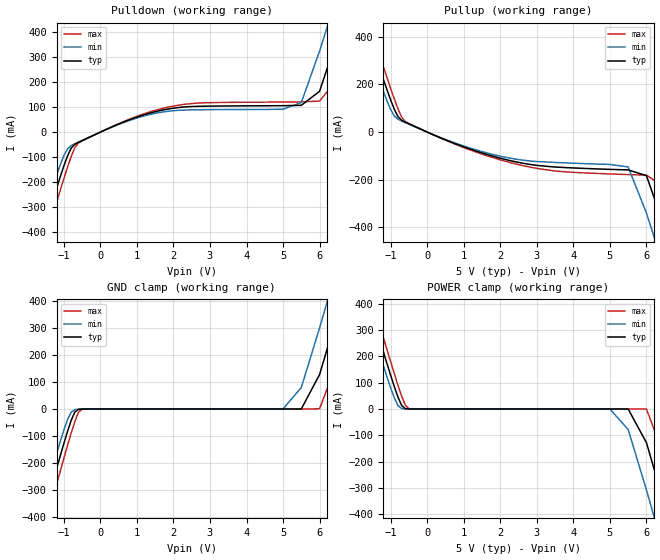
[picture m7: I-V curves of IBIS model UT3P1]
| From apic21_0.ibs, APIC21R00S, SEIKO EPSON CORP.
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[Model]   UT3P1
Model_type   I/O
Polarity   Non-Inverting
Vinh=2.0V
Vinl=0.8V
|   typ   min   max
C_comp   0   NA   NA
|   typ   min   max
[Voltage range]   5.0   4.5   5.5
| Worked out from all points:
|   slope of the pulldown table from 0 to 0.75 V, typ, clamps not added: 16 ohm
|   slope of the pullup table from 0 to 0.75 V, typ, clamps not added: 15.7 ohm
|   GND clamp passes 1 mA (typ) near -0.57 V on its own axis
|   POWER clamp passes 1 mA (typ) near -0.60 V on its own axis
[Pulldown]
|   Voltage   I(typ)   I(min)   I(max)
-10V      -4.641A    -4.561A    -4.722A
-1.8V     -515.6mA   -455.4mA   -577.1mA
-1.5V     -369.1mA   -311.5mA   -428.5mA
-1V       -136.2mA   -94.65mA   -186.9mA
-700mV    -49.13mA   -46.7mA    -62.65mA
-500mV    -34.39mA   -33.13mA   -35.47mA
2V        95.71mA    85.62mA    104.2mA
5.5V      107.2mA    118.1mA    121.1mA
6V        163.3mA    324.3mA    124.1mA
6.5V      383.2mA    554.6mA    215.7mA
7V        616.7mA    789.2mA    443.8mA
10V       2.052A     2.22A      1.883A
[Pullup]
|   Voltage   I(typ)   I(min)   I(max)
-10V      4.425A     4.351A     4.501A
-1.9V     543.7mA    486.7mA    601.8mA
-1.6V     403.5mA    348.5mA    460mA
-1V       134.3mA    94.05mA    182.5mA
-700mV    49.18mA    46.55mA    62.69mA
-500mV    34.58mA    33.18mA    35.77mA
2.5V      -127.1mA   -115.2mA   -136.4mA
5.5V      -158.7mA   -146.1mA   -178.2mA
6V        -182.8mA   -339.7mA   -180.3mA
6.5V      -401.8mA   -579.5mA   -231.7mA
7V        -645.5mA   -825.1mA   -465.2mA
10V       -2.147A    -2.323A    -1.97A
[GND_clamp]
|   Voltage   I(typ)   I(min)   I(max)
-10V      -4.641A    -4.561A    -4.722A
-1.7V     -464.4mA   -404.1mA   -526mA
-1.5V     -366.4mA   -307.5mA   -426.8mA
-1.4V     -317.7mA   -259.7mA   -377.4mA
-900mV    -83.36mA   -39.48mA   -135.4mA
-500mV    -283.5uA   -329.1uA   -653.3uA
5V        319.4pA    38.04uA    -10uA
5.5V      47.76uA    79.28mA    300.3pA
6V        127.1mA    299.3mA    663.8uA
6.5V      354.7mA    531.1mA    178.7mA
7V        589.3mA    766.1mA    411.3mA
10V       2.021A     2.194A     1.847A
[POWER_clamp]
|   Voltage   I(typ)   I(min)   I(max)
-10V      4.425A     4.35A      4.5A
-1.8V     495mA      437.8mA    553.3mA
-1.6V     401.3mA    345.2mA    458.5mA
-1.5V     354.7mA    299.3mA    411.4mA
-900mV    84.31mA    41.36mA    133.6mA
-500mV    47.76uA    38.04uA    664.9uA
5V        -100uA     -329.1uA   -100uA
5.5V      -283.5uA   -77.93mA   -110uA
6V        -127.9mA   -307.3mA   -653.1uA
6.5V      -366.3mA   -550.6mA   -182.6mA
7V        -612.6mA   -797.4mA   -426.8mA
10V       -2.117A    -2.297A    -1.935A
[Ramp]
|   V_typ   V_min   V_max
dV/dt_r   3.00/3.201e-10   2.70/3.277e-10   3.30/3.248e-10
dV/dt_f   3.00/3.830e-10   2.70/3.713e-10   3.30/3.864e-10
R_load = 5000ohm
